VAR_GLOBAL
	
//datapoints SLAVE -> MASTER (monitoring direction)
	(* Input *)

	(* Output *)
	
	(* Memory *)

	(* Data *)
		(*Single Points*)
			// bSlaveToMaster
			bSlaveToMaster		: BOOL;		//  obj addr: 10 - M_SP_NA_1
			nSIQ_bSlaveToMaster	: BYTE;		// data value and qualifier				
			eSPI_bSlaveToMaster	: E_IEC870_5_101SPI; // data value as enum type
			nQDS_bSlaveToMaster	: BYTE;		// data qualifier
		
		
//datapoints MASTER -> SLAVE (control direction)
	(* Input *)

	(* Output *)
	
	(* Memory *)

	(* Data *)
		(*Single Commands*)
			// bMasterToSlave
			bMasterToSlave		: BOOL;		// obj addr: 101 - C_SC_NA_1
			nSCO_bMasterToSlave	: BYTE;		// data value and qualifier
			eSCS_bMasterToSlave	: E_IEC870_5_101SCS; // data value as enum type
			eQU_bMasterToSlave	: E_IEC870_5_101QU; // data qualifier
	

//other variables

END_VAR
